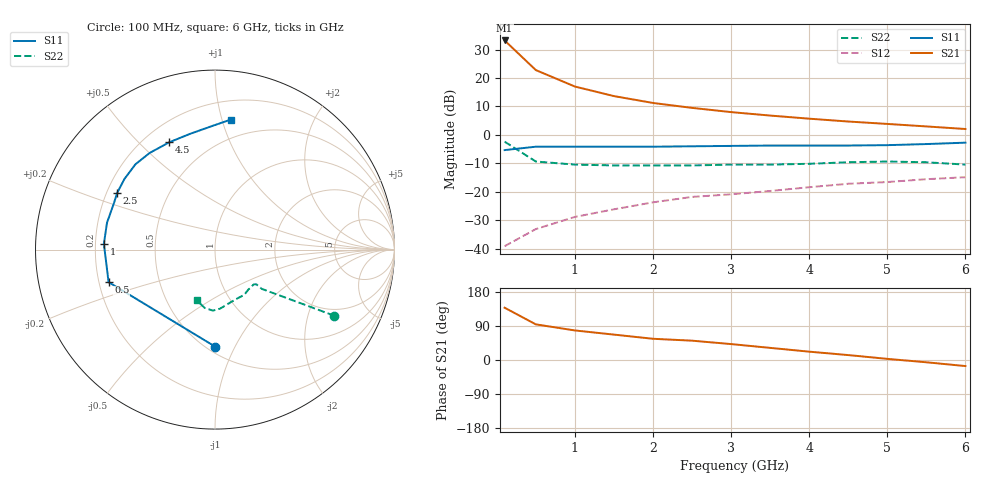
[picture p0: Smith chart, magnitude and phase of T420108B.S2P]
!AT-42010
!S-PARAMETERS at Vce=8V  Ic=35mA.  LAST UPDATED 07-21-92
# ghz s ma r 50
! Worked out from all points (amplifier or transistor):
!   13 points, 100 MHz to 6 GHz, reference 50 ohm
!   highest |S21| = 33.2 dB at 100 MHz (marker M1)
!   |S21| within 3 dB of that: start of sweep to 215 MHz
!   unconditionally stable (mu >= 1): 905.7 MHz to 5.127 GHz
!   at 1 GHz: K = 1.04, MAG = 21.8 dB, |S12| = -28.9 dB
!   at 3 GHz: K = 1.12, MAG = 12.4 dB, |S12| = -20.9 dB
!   at 6 GHz: K = 0.88, MSG = 8.5 dB, |S12| = -14.9 dB
!   S11 on the Smith chart (normalised r, x): 100 MHz: 0.55, -0.84; 500 MHz: 0.24, -0.14; 1 GHz: 0.23, +0.02; 2.5 GHz: 0.24, +0.25; 4.5 GHz: 0.30, +0.62; 6 GHz: 0.34, +1.07
0.1  0.54 -90.0  45.97 138.0  0.011 54.0  0.76 -29.0
0.5  0.62 -163.0  13.83 94.0  0.022 52.0  0.34 -40.0
1  0.62 177.0  7.1 78.0  0.036 59.0  0.3 -40.0
1.5  0.62 166.0  4.82 67.0  0.049 61.0  0.29 -42.0
2  0.62 155.0  3.65 56.0  0.065 57.0  0.29 -47.0
2.5  0.63 150.0  2.99 51.0  0.081 62.0  0.29 -50.0
3  0.64 142.0  2.52 42.0  0.09 63.0  0.3 -57.0
3.5  0.65 133.0  2.19 32.0  0.103 59.0  0.3 -67.0
4  0.65 124.0  1.93 22.0  0.12 54.0  0.31 -76.0
4.5  0.65 113.0  1.72 13.0  0.138 49.0  0.33 -85.0
5  0.66 102.0  1.56 3.0  0.148 45.0  0.34 -92.0
5.5  0.69 91.0  1.41 -6.0  0.166 39.0  0.33 -100.0
6  0.73 83.0  1.27 -16.0  0.18 32.0  0.3 -110.0
